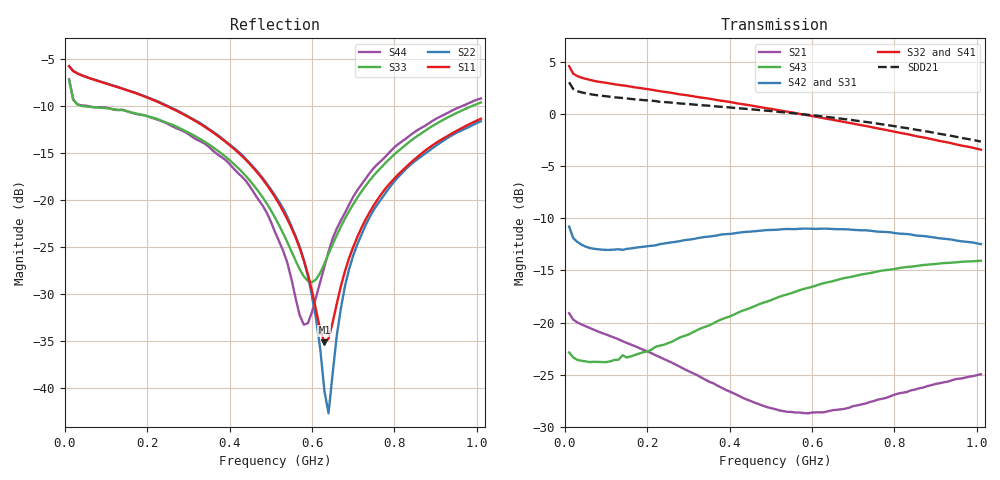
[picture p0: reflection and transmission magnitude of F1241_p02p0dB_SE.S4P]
! Integrated Device Technology
! Corporate Headquarters
! 6024 Silver Creek Valley Road
! San Jose, CA 95138  USA
! Phone:  1-408-284-8200
! Toll Free:  1-800-223-1366
! Webpage:  http://www.idt.com/
! Timing and RF Division
! 515 Groton Road, Suite 102
! Westford, MA 01886-6024
! Device:  F1241
! Description: Dual Intermediate Frequency Digital Variable Gain Amplifier
! Frequency:  10.0 -  500.00 MHz
! Package:  5x5 mm QFN Plastic Package: 32 pin
! Ports:  8 RF, 20 DC
!  Pin  1  = GA3  Pin 17  = RF OUT_B+
!  Pin  2  = GA4  Pin 18  = RF OUT_B-
!  Pin  3  = GA5  Pin 19  = STBY_B
!  Pin  4  = ISET_A  Pin 20  = Ground
!  Pin  5  = ISET_B  Pin 21  = Ground
!  Pin  6  = GB5  Pin 22  = STB_A
!  Pin  7  = GB4  Pin 23  = RF OUT_A-  = Port 4
!  Pin  8  = GB3  Pin 24  = RF OUT_A+  = Port 3
!  Pin  9  = GB2  Pin 25  = NO CONNECT
!  Pin 10  = GB1  Pin 26  = NO CONNECT
!  Pin 11  = RF IN_B+  Pin 27  = VCC
!  Pin 12  = RF IN_B-  Pin 28  = Ground
!  Pin 13  = Ground  Pin 29  = RF IN_A-  = Port 2
!  Pin 14  = VCC  Pin 30  = RF IN_A+  = Port 1
!  Pin 15  = NO CONNECT  Pin 31  = GA1
!  Pin 16  = NO CONNECT  Pin 32  = GA2
! State:  18
! Gain State:  2.0 dB
! Voltages:  Vcc = +5.00 Volts  Icc approximately 160.0 mA or 80 mA per channel.
! Data:  The device was measured on a custom evaluation board which has
!  individual transmission lines to the RF pins.  Data was collected
!  using a calibrated network analyzer.  The evaluation board was
!  de-embedded using a port reference technique.
!  The reference plane is the edge of the package pin.
!  Only Channel A was measured.
!  This data is in single-ended operation.  If your needs are balanced
!  or differential S-parameters then this file needs to be used a
!  linear simulator.
! Misc:  Lot Code  160028MY
!  Action Tracker AT004
! Date Measured:  2014-08-14
! Date:  2014-08-28  MJV
! Note:
!  Integrated Device Technology supplies this data as a sample of measured
!  data at the package pin for this product.  Your particular data for this
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# Hz S dB R 50
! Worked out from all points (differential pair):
!   101 points, 10 MHz to 1.01 GHz, reference 50 ohm
!   strongest paths, dB at 10 MHz, 260 MHz, 510 MHz, 760 MHz, 1.01 GHz:
!     S32: 4.6, 2.0, 0.4, -1.4, -3.4
!     S41: 4.6, 2.0, 0.4, -1.5, -3.6
!     S42: -10.8, -12.3, -11.1, -11.3, -12.5
!     S31: -10.8, -12.3, -11.1, -11.4, -12.6
!     S43: -22.9, -21.8, -17.7, -15.1, -14.1
!     S21: -19.1, -23.9, -28.3, -27.4, -25.0
!   taken as a pair (ports 2,1 in; 3,4 out), SDD21 dB: 3.1, 1.1, 0.3, -0.9, -2.6
!   lowest |S11| = -35.2 dB at 630 MHz (marker M1), VSWR 1.04, Z = 48.9 - j1.29 ohm
!   |S11| at or under -10 dB: 245 MHz to end of sweep
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1e7  -5.80 -12.6  -19.10 -16.7  -37.54 1.1  -20.23 11.4
     -19.10 -16.7  -5.80 -12.4  -20.25 11.1  -37.55 1.5
     -10.78 159.8  4.61 171.8  -7.26 -32.9  -22.95 -175.8
     4.65 171.9  -10.78 159.9  -22.87 -175.7  -7.19 -32.9
2.5e8  -10.10 -29.8  -23.68 -28.7  -35.89 21.5  -20.95 -16.0
       -23.68 -29.0  -10.05 -27.7  -20.90 -15.9  -35.81 21.0
       -12.35 85.5  2.11 138.1  -11.86 -23.0  -22.08 133.0
       2.08 137.4  -12.35 85.6  -21.98 132.6  -11.95 -21.7
4.7e8  -17.27 -47.8  -27.70 -21.3  -32.57 19.2  -20.85 -29.5
       -27.83 -22.4  -17.14 -42.2  -20.70 -28.9  -32.55 17.3
       -11.26 33.6  0.71 109.5  -19.14 -48.4  -18.50 100.0
       0.65 108.5  -11.20 33.0  -18.26 99.8  -20.01 -43.3
5.8e8  -26.48 -68.3  -28.36 -8.7  -31.38 14.7  -20.90 -37.1
       -28.69 -9.0  -26.40 -52.9  -20.65 -36.7  -31.37 12.3
       -11.07 12.6  -0.04 96.3  -28.17 -105.1  -17.05 84.5
       -0.14 95.1  -10.98 11.6  -16.77 83.9  -33.30 -110.9
6.3e8  -35.17 -130.7  -28.24 -3.2  -30.90 12.2  -20.96 -40.8
       -28.60 -2.8  -40.35 -96.3  -20.66 -40.3  -30.85 9.7
       -11.09 4.0  -0.39 90.5  -26.81 -167.0  -16.48 77.6
       -0.51 89.2  -10.98 2.7  -16.20 77.1  -27.12 166.8
7.5e8  -20.59 136.8  -27.30 6.0  -29.81 5.9  -21.21 -49.6
       -27.53 7.3  -21.07 132.2  -20.80 -49.2  -29.82 2.8
       -11.34 -14.8  -1.28 77.0  -17.42 150.1  -15.40 61.9
       -1.44 75.8  -11.23 -16.8  -15.18 61.5  -16.62 141.6
1.01e9  -11.39 120.9  -25.02 9.3  -28.26 -11.3  -22.23 -66.8
        -24.96 10.8  -11.66 120.4  -21.57 -67.0  -28.19 -14.8
        -12.62 -46.6  -3.41 50.8  -9.66 129.1  -14.32 32.4
        -3.64 49.8  -12.47 -49.7  -14.07 32.1  -9.23 125.0
